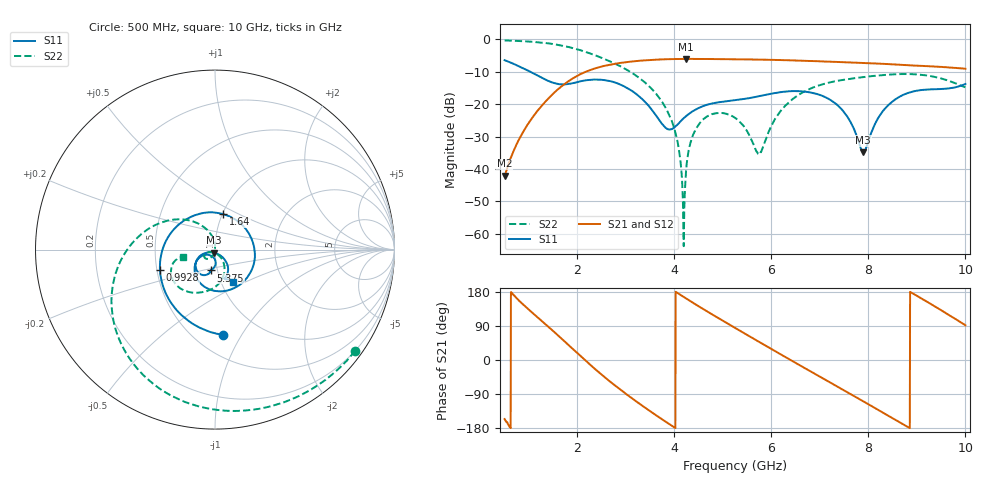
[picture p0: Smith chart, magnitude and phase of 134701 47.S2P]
!  2-Port S-parameters saved by WinCal
! VAR MeasName=S-Parameters (CALIBRATED_DATA) read from VNA (N5242A)
! VAR MeasDate=2013-7-3 16:38:25
! VAR NAME=134701 47
! VAR FILENAME=134701 47.S2P
! VAR DATE=2013-7-3 16:38:25
! VAR PHYS_PORTS=1,2
# Hz S MA R 50
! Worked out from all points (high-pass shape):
!   1601 points, 500 MHz to 10 GHz, reference 50 ohm
!   highest |S21| = -6.02 dB at 4.235 GHz (marker M1); lowest = -42.1 dB at 500 MHz (marker M2)
!   |S21| within 3 dB of the highest: 2.352 GHz to 9.952 GHz (7.601 GHz wide, 124 % of centre)
!   lowest |S11| = -34.9 dB at 7.892 GHz (marker M3), VSWR 1.04, Z = 49.4 - j1.7 ohm
!   |S11| at or under -10 dB: 1.031 GHz to end of sweep
!   |S22| runs from -63.8 to -0.3 dB; largest |S21 - S12| = 0.0021
!   S11 on the Smith chart (normalised r, x): 500 MHz: 0.68, -0.84; 992.8 MHz: 0.52, -0.13; 1.64 GHz: 1.01, +0.42; 5.375 GHz: 0.93, -0.22; 10 GHz: 1.13, -0.43
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5e8  0.4776 -84.6  0.007832 -155.8  0.007888 -154.9  0.9628 -35.9
9.928125e8  0.3269 -159.7  0.0508 133.5  0.05079 133.3  0.9256 -70.8
1.64e9  0.2029 77.2  0.1798 60.4  0.1795 60.3  0.8142 -117.3
2.085312e9  0.2274 -13.7  0.2958 8.0  0.2954 7.9  0.6721 -148.5
2.940312e9  0.1926 -120.6  0.4386 -83.5  0.4381 -83.5  0.3666 158.8
3.670625e9  0.0594 -150.7  0.4894 -150.0  0.4888 -149.9  0.1304 114.3
4.026875e9  0.0457 -99.9  0.4973 179.9  0.4973 179.9  0.03509 92.0
4.104062e9  0.05186 -92.4  0.4978 173.6  0.4978 173.6  0.0174 88.7
4.18125e9  0.05964 -88.8  0.4991 167.2  0.4986 167.3  0.002042 107.6
4.234688e9  0.06458 -88.1  0.4999 162.9  0.4995 162.9  0.008216 -101.9
4.311875e9  0.07193 -87.2  0.4992 156.8  0.4992 156.8  0.02221 -105.8
4.507812e9  0.08778 -89.1  0.4989 141.3  0.4991 141.3  0.04903 -117.5
5.25e9  0.1153 -100.0  0.4927 84.7  0.493 84.7  0.06171 -154.9
5.374688e9  0.1185 -100.6  0.4909 75.5  0.4915 75.4  0.05115 -158.8
5.754688e9  0.1332 -103.3  0.4873 47.2  0.4875 47.2  0.01732 -103.0
6.2e9  0.1534 -112.2  0.4796 14.4  0.4798 14.4  0.07999 -55.6
6.835312e9  0.1498 -134.9  0.4637 -32.0  0.4634 -32.1  0.1778 -79.4
7.452812e9  0.0827 -158.7  0.4459 -77.0  0.4458 -77.0  0.236 -101.0
7.892188e9  0.01799 -107.2  0.4326 -108.9  0.4319 -108.9  0.2616 -113.2
8.420625e9  0.09824 -48.9  0.4149 -147.9  0.4138 -147.9  0.2857 -127.8
9.133125e9  0.1664 -69.7  0.3887 159.4  0.3886 159.5  0.2816 -150.0
1e10  0.2052 -61.5  0.3522 91.7  0.3523 91.9  0.1819 -166.7
